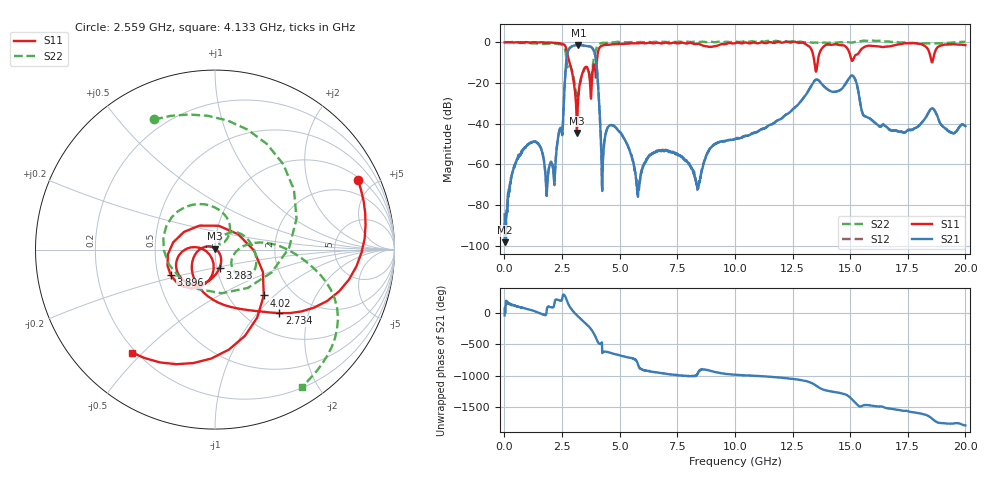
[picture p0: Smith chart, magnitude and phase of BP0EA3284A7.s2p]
! 9/17/2020 12:45:23 PM
! C:\ANRITSUVNA\DATA\MLO\SAMPLES\RAYTHEOM BP\17365_20GH_91720 .S2P
! CHANNEL.1
! TR.MEASUREMENT
! CORRECTED.DATA
# GHZ S RI R 50.0
! FREQ.GHZ  S11RE  S11IM  S31RE  S31IM  S13RE  S13IM  S33RE  S33IM
!; PortSelection: Port_13
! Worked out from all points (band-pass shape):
!   1601 points, 10 MHz to 20 GHz, reference 50 ohm
!   highest |S21| = -1.43 dB at 3.208 GHz (marker M1); lowest = -98.3 dB at 22.49 MHz (marker M2)
!   |S21| within 3 dB of the highest: 2.757 GHz to 3.888 GHz (1.131 GHz wide, 34 % of centre)
!   lowest |S11| = -44.6 dB at 3.146 GHz (marker M3), VSWR 1.01, Z = 50.1 + j0.585 ohm
!   |S11| at or under -10 dB: 2.831 GHz to 4.012 GHz (1.181 GHz wide, 34.5 % of centre); 13.45 GHz to 13.59 GHz (132.3 MHz wide, 0.978 % of centre)
!   |S22| runs from -27.9 to 0.8 dB; largest |S21 - S12| = 0.0029
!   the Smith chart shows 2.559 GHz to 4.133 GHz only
!   S11 on the Smith chart (normalised r, x): 2.559 GHz: 1.13, +4.07; 2.734 GHz: 1.39, -1.32; 3.283 GHz: 1.03, -0.21; 3.896 GHz: 0.58, -0.18; 4.02 GHz: 1.45, -0.86; 4.133 GHz: 0.18, -0.46
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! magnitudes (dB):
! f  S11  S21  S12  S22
! 10 MHz  -0.2  -84.6  -88.6  0.0
! 22.49 MHz  -0.1  -98.3  -92.6  0.0
! 1.047 GHz  -0.1  -50.2  -50.0  -0.3
! 2.146 GHz  -0.3  -66.8  -66.1  -0.6
! 2.559 GHz  -1.0  -34.0  -34.0  -1.9
! 2.734 GHz  -6.0  -5.4  -5.4  -12.4
! 3.146 GHz  -44.6  -1.5  -1.5  -27.4
! 3.208 GHz  -26.6  -1.4  -1.4  -26.1
! 3.283 GHz  -19.7  -1.5  -1.5  -20.2
! 3.346 GHz  -16.7  -1.5  -1.5  -16.9
! 3.896 GHz  -10.9  -4.6  -4.6  -7.2
! 4.02 GHz  -8.6  -13.9  -13.8  -2.1
! 4.133 GHz  -2.6  -34.6  -34.6  -0.9
! 4.27 GHz  -1.6  -59.2  -58.4  -0.4
! 5.795 GHz  -0.6  -76.0  -74.9  0.0
! 6.682 GHz  -0.3  -53.3  -53.3  0.0
! 8.393 GHz  -0.9  -72.0  -71.2  0.0
! 10.01 GHz  -0.5  -47.7  -47.5  0.3
! 13.34 GHz  -4.2  -20.9  -20.9  -0.3
! 15.11 GHz  -9.0  -16.6  -16.5  -0.2
! 16.68 GHz  -2.1  -42.5  -42.6  0.3
! 20 GHz  -1.5  -41.2  -41.2  0.2
